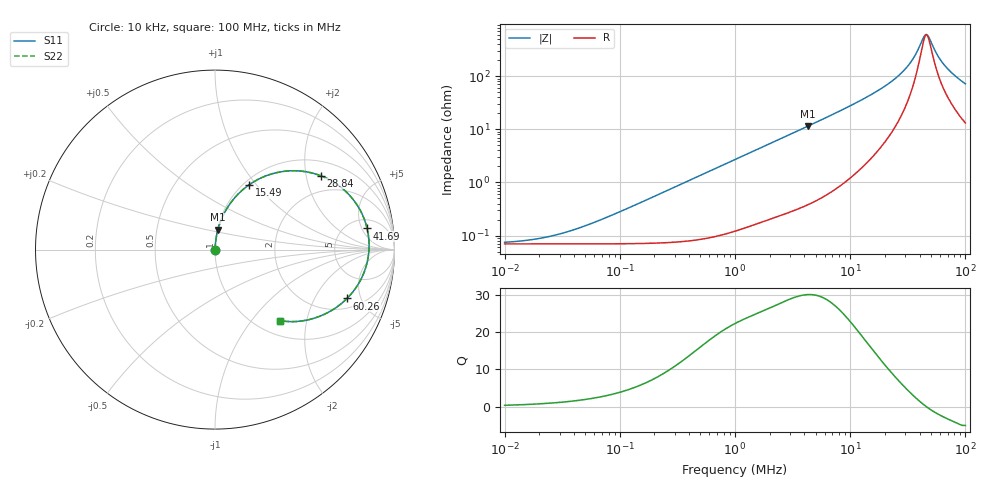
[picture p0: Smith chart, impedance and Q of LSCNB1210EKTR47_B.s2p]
! LSCNB1210EKTR47_B  S-PARAMETER MODEL  ( Standard Model )
! Model Generated by TAIYO YUDEN Corporation (http://www.ty-top.com)
! Version 1.0
! TAIYO YUDEN Control No. 191108
! Copyright(c) 2019 TAIYO YUDEN CO.,LTD. All Rights Reserved.
! Product Description (link to TY-COMPAS)
! https://ds.yuden.co.jp/TYCOMPAS/or/detail?pn=LSCNB1210EKTR47MB&u=M
! Products Name : Inductors
! Characteristics :
!  Inductance : 0.47 [uH] , SRF(min) : - [Hz] , DC Resistance(max) : 82 [mOhm]
!  Rated Current : Saturation  2.3 [A] (dL = 30 [%]), Temp Rise  1.6 [A] (dT = 40 [degC])
!  Case Size : 1.25 x 1.05 / 0.049 x 0.041 [mm/inch] , Thickness : 0.5 / 0.02 [mm/inch]
!  (Conditions: Temperature = 25 [degC] , DC Bias Current = 0 [A])
! External Node Assignments :
!  1  o---GGG---o  2
! GND o---------o GND
! Frequency Range : 10kHz  -  100MHz  [ 402 STEP ]
# MHz S RI R 50
! Freq[MHz].  S11 Real  S11 Imag  S21 Real  S21 Imag  S12 Real  S12 Imag  S22 Real  S22 Imag
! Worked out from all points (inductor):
!   401 points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, 10 kHz to 100 MHz, reference 50 ohm
!   read as one part in series: L = 434 nH near 77.62 kHz
!   highest Q = 30 at 4.266 MHz (marker M1), where L = 424 nH
!   self-resonance near 45.97 MHz
!   S11 on the Smith chart (normalised r, x): 10 kHz: 1.00, +0.00; 15.49 MHz: 1.06, +0.92; 28.84 MHz: 1.43, +2.43; 41.69 MHz: 7.22, +6.35; 60.26 MHz: 2.67, -3.78; 100 MHz: 1.26, -1.40
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0.01  0.0007 0.000272  0.9993 -0.000272  0.9993 -0.000272  0.0007 0.000272
0.022387  0.0007 0.000609  0.9993 -0.000609  0.9993 -0.000609  0.0007 0.000609
0.046774  0.000702 0.00127  0.9993 -0.00127  0.9993 -0.00127  0.000702 0.00127
0.087096  0.000708 0.00237  0.9993 -0.00237  0.9993 -0.00237  0.000708 0.00237
0.218776  0.000763 0.00595  0.9992 -0.00595  0.9992 -0.00595  0.000763 0.00595
1  0.00194 0.027  0.9981 -0.027  0.9981 -0.027  0.00194 0.027
4.265795  0.0164 0.1114  0.9836 -0.1114  0.9836 -0.1114  0.0164 0.1114
4.677351  0.0193 0.1218  0.9807 -0.1218  0.9807 -0.1218  0.0193 0.1218
9.549926  0.0734 0.2404  0.9266 -0.2404  0.9266 -0.2404  0.0734 0.2404
15.48817  0.189 0.3604  0.811 -0.3604  0.811 -0.3604  0.189 0.3604
21.87762  0.3668 0.4334  0.6332 -0.4334  0.6332 -0.4334  0.3668 0.4334
28.84032  0.5882 0.4119  0.4118 -0.4119  0.4118 -0.4119  0.5882 0.4119
32.35937  0.6897 0.3566  0.3103 -0.3566  0.3103 -0.3566  0.6897 0.3566
35.48134  0.7632 0.2871  0.2368 -0.2871  0.2368 -0.2871  0.7632 0.2871
41.68694  0.8476 0.1177  0.1524 -0.1177  0.1524 -0.1177  0.8476 0.1177
44.66836  0.8585 0.0346  0.1415 -0.0346  0.1415 -0.0346  0.8585 0.0346
46.77351  0.8563 -0.021  0.1437 0.021  0.1437 0.021  0.8563 -0.021
48.97788  0.8468 -0.0751  0.1532 0.0751  0.1532 0.0751  0.8468 -0.0751
52.48075  0.8204 -0.1507  0.1796 0.1507  0.1796 0.1507  0.8204 -0.1507
60.25596  0.7355 -0.2722  0.2645 0.2722  0.2645 0.2722  0.7355 -0.2722
74.13102  0.5763 -0.3742  0.4237 0.3742  0.4237 0.3742  0.5763 -0.3742
100  0.3616 -0.3957  0.6384 0.3957  0.6384 0.3957  0.3616 -0.3957
